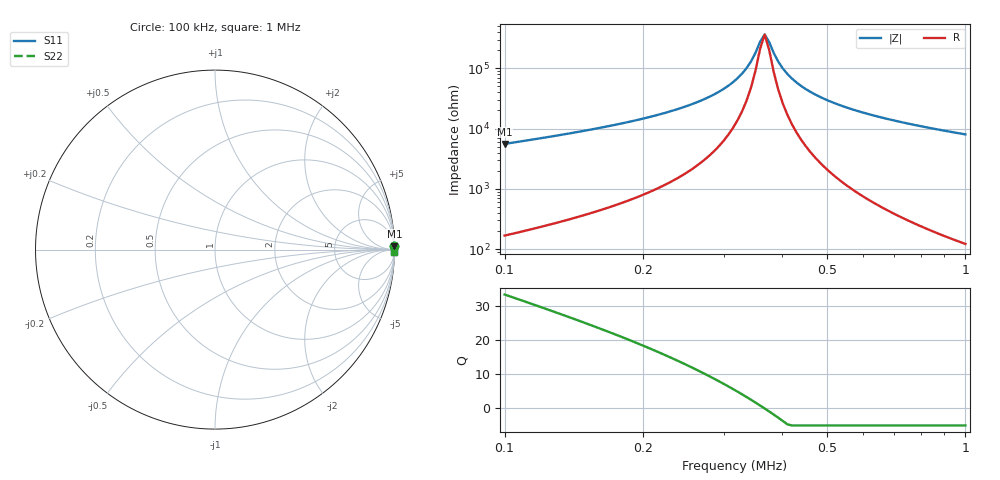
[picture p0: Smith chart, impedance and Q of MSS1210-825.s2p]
# MHz S MA R 50
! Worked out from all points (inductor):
!   102 points, 100 kHz to 1 MHz, reference 50 ohm
!   read as one part in series: L = 8.15 mH near 100 kHz
!   highest Q = 33.3 at 100 kHz (marker M1), where L = 8.85 mH
!   self-resonance near 358.5 kHz
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0.1  0.9993 1.0  0.01796 -87.3  0.01796 -87.3  0.9993 1.0
0.2546482  0.9997 0.2  0.003954 -85.0  0.003954 -85.0  0.9997 0.2
0.2919756  0.9997 0.1  0.002447 -82.7  0.002447 -82.7  0.9997 0.1
0.319853  0.9997 0.1  0.001475 -78.5  0.001475 -78.5  0.9997 0.1
0.3347746  0.9997 0.1  0.001001 -73.3  0.001001 -73.3  0.9997 0.1
0.3424944  0.9997 0.0  0.0007714 -68.4  0.0007714 -68.4  0.9997 0.0
0.3503922  0.9997 0.0  0.0005521 -59.5  0.0005521 -59.5  0.9997 0.0
0.3584722  0.9997 0.0  0.0003629 -40.2  0.0003629 -40.2  0.9997 0.0
0.3667384  0.9997 -0.0  0.0002744 1.5  0.0002744 1.5  0.9997 -0.0
0.3751953  0.9997 -0.0  0.0003681 42.5  0.0003681 42.5  0.9997 -0.0
0.3838472  0.9997 -0.0  0.000559 61.3  0.000559 61.3  0.9997 -0.0
0.3926986  0.9997 -0.0  0.0007788 70.0  0.0007788 70.0  0.9997 -0.0
0.4017542  0.9997 -0.1  0.001009 74.9  0.001009 74.9  0.9997 -0.1
0.4110185  0.9997 -0.1  0.001244 77.9  0.001244 77.9  0.9997 -0.1
0.430193  0.9997 -0.1  0.001723 81.4  0.001723 81.4  0.9997 -0.1
0.460645  0.9998 -0.1  0.002455 84.1  0.002455 84.1  0.9998 -0.1
0.5046268  0.9998 -0.2  0.003453 85.9  0.003453 85.9  0.9998 -0.2
0.5528079  0.9998 -0.3  0.004482 86.8  0.004482 86.8  0.9998 -0.3
0.6195541  0.9998 -0.3  0.005823 87.5  0.005823 87.5  0.9998 -0.3
0.7103709  0.9998 -0.4  0.007534 88.0  0.007534 88.0  0.9998 -0.4
0.8524974  0.9998 -0.6  0.01004 88.3  0.01004 88.3  0.9998 -0.6
1  0.9997 -0.7  0.01251 88.4  0.01251 88.4  0.9997 -0.7
